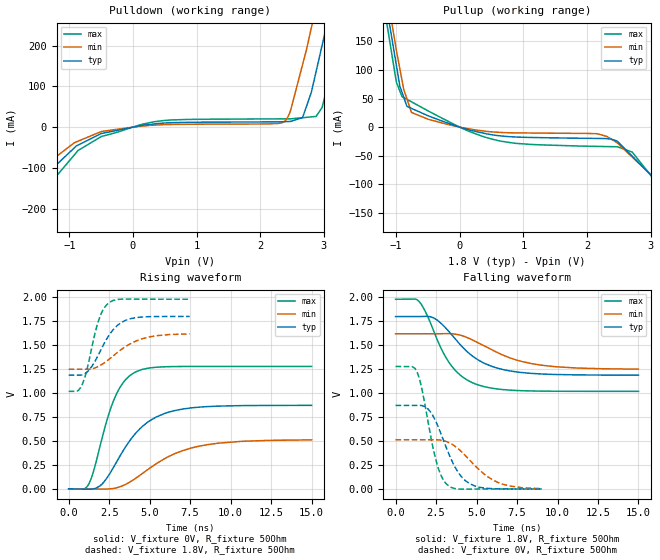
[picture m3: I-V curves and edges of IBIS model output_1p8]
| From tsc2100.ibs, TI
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|   output_1p8 Model
[Model]   output_1p8
Model_type   Output
Polarity   Non-Inverting
Vmeas = 0.9
Vref = 0.9
Cref = 10pF
Rref = 50
|   typ   min   max
|   (nom PVT)   (fast PVT)   (slow PVT)
|C_comp from frequency sweep method (F=13MHz)
|C_comp   3.972e-12   3.646e-12   4.140e-12
|ON state : BUFFER OUTPUT TURNED HIGH
|C_comp   3.972e-12   3.646e-12   4.140e-12
|OFF state: BUFFER OUTPUT TURNED LOW
|C_comp   2.841e-12   2.717e-12   2.929e-12
|C_comp from LC tank measurement(L=1nH)
|Resonant Frequency(Hz)   4.160e+09   4.190e+09   4.110e+09
C_comp   1.465e-12   1.444e-12   1.501e-12
|ON state : BUFFER OUTPUT TURNED HIGH
|Resonant Frequency(Hz)   4.160e+09   4.190e+09   4.110e+09
|C_comp   1.465e-12   1.444e-12   1.501e-12
|OFF state: BUFFER OUTPUT TURNED LOW
|Resonant Frequency(Hz)   4.270e+09   4.271e+09   4.267e+09
|C_comp   1.391e-12   1.390e-12   1.392e-12
| Where nom  PVT is Nominal Process, 1.8V, 26C
|   Fast PVT is Strong Process,  1.98V, -40C
|   Slow PVT is Weak Process,   1.62V, 86C
[Voltage Range]   1.8   1.62   1.98
|Ambient Temperature   25   85   -40
|Junction Temperature
[Temperature Range]   26   86   -40
[Pullup Reference]   1.8   1.62   1.98
[Pulldown Reference]   0   0   0
[Power Clamp Reference]   1.8   1.62   1.98
[GND Clamp Reference]   0   0   0
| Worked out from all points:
|   slope of the pulldown table from 0 to 0.27 V, typ, clamps not added: 40.6 ohm
|   slope of the pullup table from 0 to 0.27 V, typ, clamps not added: 33.8 ohm
|   falling waveform, V_fixture 1.8V, R_fixture 50Ohm: 20-80 % time 2.39ns typ, 3.09ns min, 1.83ns max; typ from 1.8 V to 1.19 V
|   rising waveform, V_fixture 0V, R_fixture 50Ohm: 20-80 % time 2.3ns typ, 3.17ns min, 1.4ns max; typ from 0 V to 0.872 V
|   rising waveform, V_fixture 1.8V, R_fixture 50Ohm: 20-80 % time 1.29ns typ, 1.91ns min, 834ps max; typ from 1.19 V to 1.8 V
|   falling waveform, V_fixture 0V, R_fixture 50Ohm: 20-80 % time 1.36ns typ, 1.98ns min, 915ps max; typ from 0.872 V to 0 V
[Pulldown]
|   Voltage   I(typ)   I(min)   I(max)
-1.8V     -259.2mA   -143.5mA   -379.3mA
-1.559V   -145.3mA   -114.7mA   -197mA
-861.3mV  -44.11mA   -34.47mA   -57.35mA
-495mV    -15.54mA   -10.71mA   -22.99mA
2.354V    13.2mA     11.18mA    20.29mA
2.479V    14.11mA    40.85mA    20.41mA
2.668V    23.63mA    153.9mA    23.17mA
2.806V    86.32mA    244.9mA    25.2mA
2.879V    136mA      296mA      26.27mA
3.091V    280.5mA    447.8mA    122.9mA
3.24V     389.9mA    556.9mA    226.4mA
3.6V      660.4mA    819.8mA    498.5mA
[Pullup]
|   Voltage   I(typ)   I(min)   I(max)
-1.8V     697.5mA    715.2mA    686.1mA
-1.132V   198.6mA    226.1mA    171.9mA
-995.9mV  107.7mA    133.9mA    78.6mA
-941.4mV  71.61mA    101.7mA    63.04mA
-829.8mV  36.23mA    49.11mA    48.52mA
-758.2mV  32.69mA    25.65mA    44.17mA
601.9mV   -14.74mA   -8.989mA   -23.42mA
2.462V    -23.83mA   -26.38mA   -34.27mA
2.711V    -50.8mA    -52.22mA   -43.55mA
3.24V     -118.6mA   -113.1mA   -127.8mA
3.479V    -173.8mA   -143.6mA   -172.1mA
3.6V      -251mA     -159mA     -221.6mA
[Ramp]
R_load = 50
|   typ   min   max
dV/dt_r   0.523348/2.29736e-09   0.307206/3.15479e-09   0.767233/1.39313e-09
dV/dt_f   0.367077/2.39111e-09   0.221497/3.08411e-09   0.576588/1.82782e-09
[Falling Waveform]
V_fixture = 1.8V
V_fixture_min = 1.62V
V_fixture_max = 1.98V
R_fixture = 50Ohm
|   Time   V(typ)   V(min)   V(max)
0s        1.8V       1.62V      1.98V
1.447ns   1.8V       1.62V      1.959V
1.846ns   1.802V     1.62V      1.85V
2.352ns   1.786V     1.62V      1.651V
3.319ns   1.639V     1.621V     1.317V
4.047ns   1.496V     1.603V     1.181V
4.954ns   1.363V     1.539V     1.095V
6.345ns   1.259V     1.42V      1.043V
8.344ns   1.207V     1.31V      1.023V
15ns      1.188V     1.251V     1.019V
[Rising Waveform]
V_fixture = 0V
V_fixture_min = 0V
V_fixture_max = 0V
R_fixture = 50Ohm
|   Time   V(typ)   V(min)   V(max)
0s        1.042nV    7.529nV    577pV
1.236ns   -2.463mV   -98.3uV    49.01mV
1.511ns   231.9uV    -767uV     169.9mV
2.035ns   46.84mV    -1.904mV   512.3mV
2.801ns   235.1mV    6.248mV    933.2mV
3.389ns   405.6mV    37.21mV    1.115V
4.099ns   573.9mV    106.7mV    1.218V
5.937ns   788.3mV    317.3mV    1.275V
8.111ns   854.2mV    448.1mV    1.279V
15ns      872.2mV    512mV      1.279V
[Rising Waveform]
V_fixture = 1.8V
V_fixture_min = 1.62V
V_fixture_max = 1.98V
R_fixture = 50Ohm
|   Time   V(typ)   V(min)   V(max)
0s        1.188V     1.249V     1.019V
532ps     1.188V     1.249V     1.022V
813ps     1.189V     1.249V     1.082V
1.091ns   1.214V     1.248V     1.22V
1.829ns   1.397V     1.278V     1.748V
2.472ns   1.599V     1.35V      1.942V
3.046ns   1.711V     1.429V     1.978V
3.867ns   1.779V     1.521V     1.981V
5.326ns   1.799V     1.597V     1.98V
7.47ns    1.8V       1.618V     1.98V
[Falling Waveform]
V_fixture = 0V
V_fixture_min = 0V
V_fixture_max = 0V
R_fixture = 50Ohm
|   Time   V(typ)   V(min)   V(max)
0s        872.5mV    513.8mV    1.279V
1.324ns   872.5mV    513.9mV    1.223V
1.632ns   870.5mV    513.9mV    1.04V
2.027ns   831.3mV    513.8mV    684mV
2.561ns   677mV      513.7mV    259.2mV
3.205ns   402.3mV    490.8mV    42.82mV
4.01ns    140.6mV    398.9mV    -1.513mV
4.884ns   31.76mV    247mV      -693.2uV
6.433ns   1.433mV    61.08mV    74.49uV
9.038ns   48.9uV     3.393mV    62.59uV
